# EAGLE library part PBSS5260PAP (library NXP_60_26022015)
60 V, 2 A PNP/PNP low VCEsat (BISS) transistor PNP/PNP low VCEsat Breakthrough In Small Signal (BISS) transistor in a leadless medium power DFN2020-6 (SOT1118) Surface-Mounted Device (SMD) plastic package. NPN/PNP complement: PBSS4260PANP. NPN/NPN complement: PBSS4260PAN. AAL Eindhoven MK
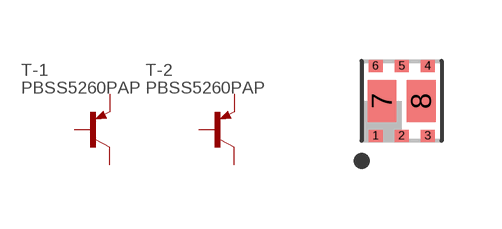
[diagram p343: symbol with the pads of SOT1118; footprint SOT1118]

Designator prefix T; gates -1=PNP -2=PNP

## PBSS5260PAP  [SOT1118]
1  -1:E  pas
2  -1:B  pas
3  -2:C  pas
4  -2:E  pas
5  -2:B  pas
6  -1:C  pas
7  -1:C  pas
8  -2:C  pas

## Footprint SOT1118 (pad centres in mm)
SOT1118 HUSON6: plastic, thermal enhanced ultra thin small outline package; no leads;6 terminals; body 2 x 2 x 0.65 mm JEDEC: -- IEC: -- JEITA: --
smd 0.35 x 0.3: 1 -0.65,-0.875; 2 0,-0.875; 3 0.65,-0.875; 4 0.65,0.875; 5 0,0.875; 6 -0.65,0.875
smd 0.72 x 1.05: 7 -0.49,0; 8 0.49,0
